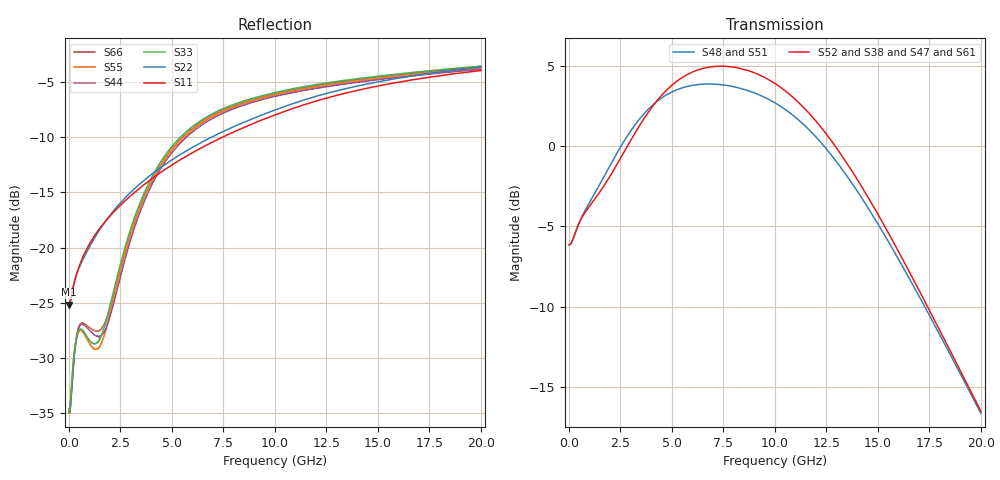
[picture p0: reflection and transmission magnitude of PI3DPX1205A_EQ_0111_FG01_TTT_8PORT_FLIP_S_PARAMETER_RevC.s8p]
! NPort=8 DATA=2000 NOISE=0 GROUPDELAY=0 COMPLEX_DATAFORMAT=POLAR
! NumOfBlock=1 NumOfParam=0
! .MODEL Smodel S TSTONEFILE=PI3DPX1205A_EQ_0111_FG01_TTT_8PORT_FLIP_S_PARAMETER_RevC.s8p TYPE=S
!  -- The above .MODEL line can be used for the S element in the netlist.
! The s parameter is extracted from the linear redriver, it is not bi-directional;
! only s(5,1)s(6,2)s(3,7)s(4,8) should be the insertion loss
!  Port definition:
!  Port1 = AIP
!  Port2 = AIN
!  Port3 = BOP
!  Port4 = BON
!  Port5 = AOP
!  Port6 = AON
!  Port7 = BIP
!  Port8 = BIN
# Hz S MA R  50
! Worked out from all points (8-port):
!   2000 points, 10 MHz to 20 GHz, reference 50 ohm
!   strongest paths, dB at 10 MHz, 5.01 GHz, 10.01 GHz, 15.01 GHz, 20 GHz:
!     S52: -6.1, 3.8, 3.9, -4.3, -16.5
!     S38: -6.1, 3.8, 3.9, -4.3, -16.5
!     S47: -6.1, 3.8, 3.9, -4.2, -16.4
!     S61: -6.1, 3.8, 3.9, -4.2, -16.4
!     S48: -6.1, 3.4, 2.7, -4.9, -16.6
!     S51: -6.1, 3.4, 2.7, -4.9, -16.6
!   lowest |S11| = -25.2 dB at 10 MHz (marker M1), VSWR 1.12, Z = 44.8 - j0.115 ohm
!   |S11| at or under -10 dB: start of sweep to 7.464 GHz
